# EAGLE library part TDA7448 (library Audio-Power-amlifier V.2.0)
The TDA7448 is a 6 channel volume controller for quality audio applications in Multi-Channels Audio Systems
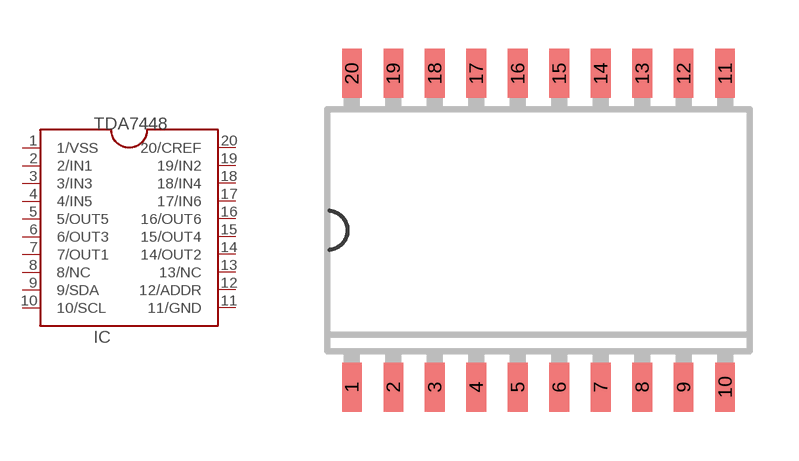
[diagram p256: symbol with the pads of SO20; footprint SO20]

Designator prefix IC

## TDA7448  [SO20]
1  1/VSS  pwr
2  2/IN1  in
3  3/IN3  in
4  4/IN5  in
5  5/OUT5  out
6  6/OUT3  out
7  7/OUT1  out
8  8/NC  nc
9  9/SDA
10  10/SCL
11  11/GND  pwr
12  12/ADDR
13  13/NC  nc
14  14/OUT2  out
15  15/OUT4  out
16  16/OUT6  out
17  17/IN6  in
18  18/IN4  in
19  19/IN2  in
20  20/CREF

## Footprint SO20 (pad centres in mm)
SO20 - Small Outline Package 7.6 x 13.0 mm
smd 0.6 x 1.5: 1 -5.715,-4.8; 2 -4.445,-4.8; 3 -3.175,-4.8; 4 -1.905,-4.8; 5 -0.635,-4.8; 6 0.635,-4.8; 7 1.905,-4.8; 8 3.175,-4.8; 9 4.445,-4.8; 10 5.715,-4.8; 11 5.715,4.8; 12 4.445,4.8; 13 3.175,4.8; 14 1.905,4.8; 15 0.635,4.8; 16 -0.635,4.8; 17 -1.905,4.8; 18 -3.175,4.8; 19 -4.445,4.8; 20 -5.715,4.8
